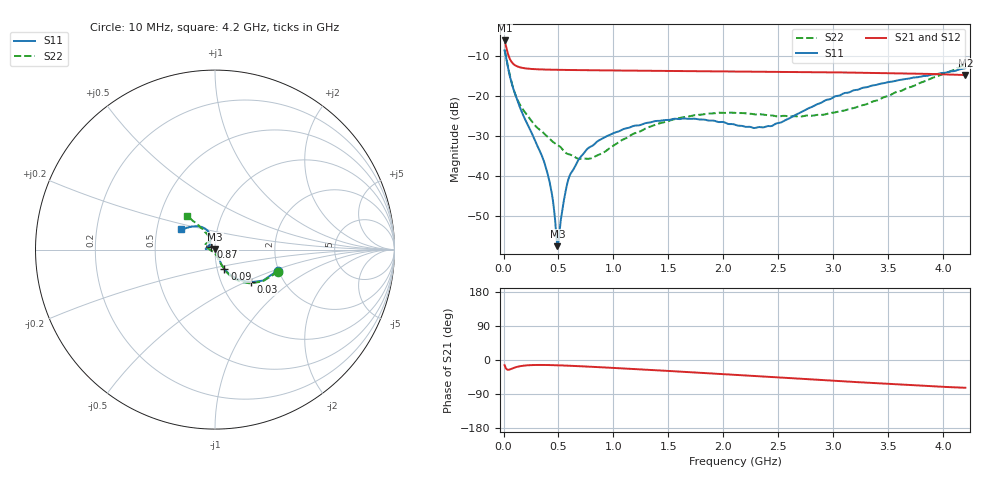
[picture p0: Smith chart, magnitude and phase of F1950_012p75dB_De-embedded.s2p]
! Integrated Device Technology
! Corporate Headquarters
! 6024 Silver Creek Valley Road
! San Jose, CA 95138  USA
! Phone:  1-408-284-8200
! Toll Free:  1-800-223-1366
! Webpage:  http://www.idt.com/
! Timing and RF Division
! 515 Groton Road, Suite 102
! Westford, MA 01886-6024
! Device:  F1950
! Description: 7-bit 0.25 dB Digital Step Attenuator
! Frequency:  150.0 -  4000.00 MHz
! Package:  4x4 mm Thin QFN Plastic Package: 24 pin
! Ports:  2 RF, 12 DC
!  Pin  1  = D0
!  Pin  2  = VDD
!  Pin  3  = Vmode
!  Pin  4  = GND
!  Pin  5  = RF1  =  Port 1
!  Pin  6  = GND
!  Pin  7  = GND
!  Pin  8  = GND
!  Pin  9  = GND
!  Pin 10  = GND
!  Pin 11  = GND
!  Pin 12  = GND
!  Pin 13  = GND
!  Pin 14  = RF2  =  Port 2
!  Pin 15  = GND
!  Pin 16  = LE
!  Pin 17  = CLK
!  Pin 18  = DATE
!  Pin 19  = D6
!  Pin 20  = D5
!  Pin 21  = D4
!  Pin 22  = D3
!  Pin 23  = D2
!  Pin 24  = D1
! State:  51
! Atten State:  12.75 dB
! Voltage:  +5.00 Volts
! Current:  Not Measured mA
! Data:  The device was measured on a the F195X evaluation board which has
!  individual transmission lines to the RF pins.  Data was collected
!  using a calibrated network analyzer.  The evaluation board was
!  de-embedded using a TRL calibration technique.
!  The reference plane is the edge of the package pin.
! Misc:  Board 2019
!  Action Tracker AT0250
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# GHz S dB R 50
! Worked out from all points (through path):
!   420 points, 10 MHz to 4.2 GHz, reference 50 ohm
!   highest |S21| = -6.24 dB at 10 MHz (marker M1); lowest = -14.9 dB at 4.2 GHz (marker M2)
!   group delay of S21, straight-line fit = 43.2 ps
!   lowest |S11| = -57.6 dB at 490 MHz (marker M3), VSWR 1.00, Z = 50.1 + j0.0715 ohm
!   |S11| at or under -10 dB: 20.41 MHz to end of sweep
!   |S22| runs from -35.8 to -8.6 dB; largest |S21 - S12| = 0.00029
!   S11 on the Smith chart (normalised r, x): 10 MHz: 1.98, -0.53; 30 MHz: 1.37, -0.54; 90 MHz: 1.08, -0.24; 870 MHz: 0.96, +0.03; 4.2 GHz: 0.67, +0.16
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0.01  -8.68 -18.5  -6.24 -13.6  -6.24 -13.6  -8.61 -19.5
0.03  -11.41 -42.6  -8.53 -24.8  -8.52 -24.8  -11.34 -44.0
0.09  -18.36 -64.1  -12.11 -21.2  -12.11 -21.2  -18.29 -64.2
0.18  -24.97 -65.3  -13.12 -15.1  -13.12 -15.1  -23.58 -70.7
0.38  -37.48 -52.9  -13.50 -13.1  -13.50 -13.2  -29.70 -76.7
0.43  -43.01 -48.0  -13.53 -13.4  -13.53 -13.4  -31.04 -79.1
0.48  -54.98 -5.9  -13.56 -13.8  -13.56 -13.8  -32.12 -85.4
0.49  -57.55 32.6  -13.57 -13.9  -13.56 -13.9  -32.27 -86.3
0.51  -53.77 98.3  -13.57 -14.1  -13.57 -14.1  -32.65 -87.3
0.55  -45.99 118.4  -13.59 -14.6  -13.59 -14.6  -33.84 -90.8
0.59  -40.86 126.6  -13.61 -15.0  -13.60 -15.0  -34.59 -99.1
0.71  -35.03 135.7  -13.64 -16.6  -13.64 -16.6  -35.73 -121.1
0.87  -31.12 144.8  -13.69 -18.9  -13.69 -18.9  -34.71 -153.3
1.1  -28.26 156.5  -13.75 -22.4  -13.75 -22.5  -30.81 -179.6
1.41  -26.30 169.3  -13.83 -27.4  -13.82 -27.5  -26.98 166.6
1.73  -25.74 176.3  -13.89 -32.7  -13.89 -32.7  -24.91 157.9
2.11  -27.33 168.4  -13.98 -39.2  -13.98 -39.3  -24.34 148.3
2.43  -27.62 135.9  -14.05 -44.6  -14.05 -44.6  -24.93 137.9
2.81  -22.75 110.3  -14.14 -51.3  -14.14 -51.3  -25.00 122.1
3.19  -18.63 112.6  -14.26 -58.0  -14.26 -58.0  -23.07 115.8
3.51  -16.58 121.3  -14.39 -63.3  -14.39 -63.3  -19.98 117.8
4.2  -13.14 148.8  -14.87 -73.3  -14.86 -73.4  -12.27 129.8
